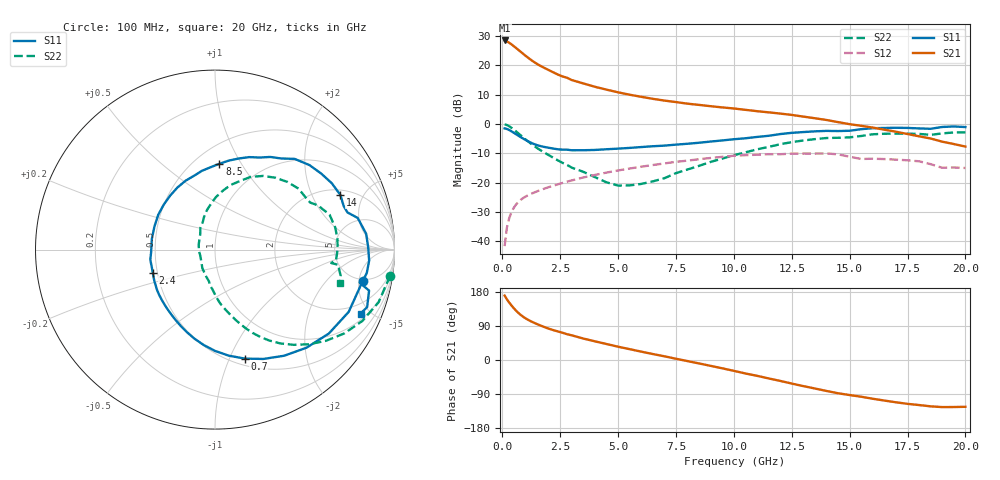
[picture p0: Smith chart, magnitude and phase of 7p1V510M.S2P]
! Infineon Technologies  Discrete & RF Semiconductors
! bfp620
! VCE =  1.5 V,  IC =  10 mA
! Common Emitter S-Parameters:  Sep 2002
# GHz  S  MA  R  50
!  f  S11  S21  S12  S22
! GHz  MAG  ANG  MAG  ANG  MAG  ANG  MAG  ANG
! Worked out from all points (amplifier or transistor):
!   59 points, 100 MHz to 20 GHz, reference 50 ohm
!   highest |S21| = 28.4 dB at 100 MHz (marker M1)
!   |S21| within 3 dB of that: start of sweep to 662 MHz
!   unconditionally stable (mu >= 1): 4.11 GHz to 10.58 GHz; 17.1 GHz to end of sweep
!   at 1 GHz: K = 0.49, MSG = 24.0 dB, |S12| = -24.8 dB
!   at 5.5 GHz: K = 1.04, MAG = 11.3 dB, |S12| = -15.2 dB
!   at 20 GHz: K = 1.37, MAG = 0.0 dB, |S12| = -15.0 dB
!   S11 on the Smith chart (normalised r, x): 100 MHz: 4.63, -5.61; 700 MHz: 0.57, -1.14; 2.4 GHz: 0.47, -0.14; 8.5 GHz: 0.65, +0.81; 14 GHz: 2.29, +3.32; 20 GHz: 1.32, -4.38
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0.1  0.8408 -12.2  26.41 170.1  0.0083 83.9  0.9862 -8.5
0.2  0.8217 -25.0  25.43 160.1  0.0173 78.3  0.9577 -17.8
0.3  0.788 -36.4  24.11 151.4  0.025 72.8  0.9125 -25.8
0.4  0.7475 -47.0  22.61 143.6  0.0318 67.9  0.8581 -33.0
0.5  0.7058 -56.9  21.08 136.4  0.0376 63.8  0.8004 -39.4
0.6  0.666 -66.2  19.58 129.9  0.0428 60.3  0.7432 -45.2
0.7  0.6292 -74.8  18.17 124.0  0.0472 57.4  0.6886 -50.4
0.8  0.5954 -82.7  16.86 118.8  0.0512 54.9  0.6377 -55.1
1  0.5359 -96.6  14.55 110.1  0.0578 51.2  0.5481 -62.6
1.3  0.4671 -113.9  11.86 100.3  0.0661 47.8  0.4428 -70.8
1.8  0.4073 -137.0  9.074 87.3  0.0787 44.4  0.3285 -81.3
2.4  0.3703 -159.3  6.941 75.4  0.0939 41.2  0.2398 -91.2
3  0.3562 -177.7  5.592 65.1  0.1093 37.8  0.1804 -100.6
3.5  0.357 170.3  4.899 56.6  0.1227 34.5  0.1531 -110.3
5  0.3801 138.6  3.459 35.1  0.1616 23.4  0.0892 -155.4
7  0.4275 105.9  2.501 9.8  0.2128 6.7  0.1191 133.6
8.5  0.4789 87.1  2.11 -9.1  0.2509 -7.7  0.1936 108.2
10.5  0.5702 64.1  1.739 -35.6  0.2943 -30.3  0.3287 82.8
13.5  0.7485 29.6  1.251 -75.2  0.3134 -64.1  0.5516 43.2
14  0.762 23.5  1.169 -81.7  0.3149 -70.7  0.5763 36.1
17  0.8611 -4.1  0.738 -111.6  0.2468 -95.1  0.6848 4.9
20  0.886 -23.7  0.412 -123.5  0.178 -106.8  0.7202 -15.0
